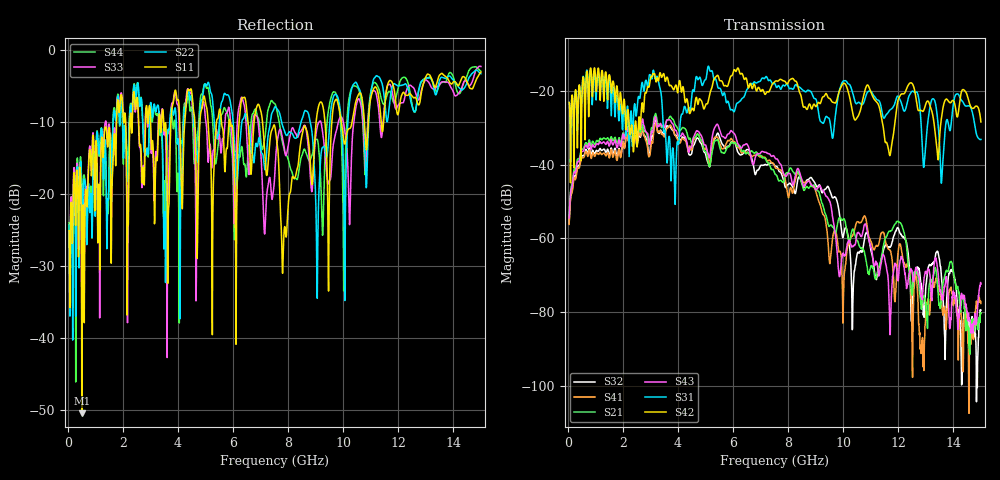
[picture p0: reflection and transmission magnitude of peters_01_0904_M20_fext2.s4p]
# MHZ S RI R 50.00
! FREQ  S11  S12  S13  S14
!  S21  S22  S23  S24
!  S31  S32  S33  S34
!  S41  S42  S43  S44
!  REAL  IMAG  REAL  IMAG  REAL  IMAG  REAL  IMAG
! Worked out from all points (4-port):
!   1496 points, 50 MHz to 15 GHz, reference 50 ohm
!   strongest paths, dB at 50 MHz, 3.79 GHz, 7.53 GHz, 11.27 GHz, 15 GHz:
!     S42: -23.1, -19.0, -17.4, -23.6, -28.4
!     S31: -23.1, -36.8, -18.2, -22.5, -33.2
!     S43: -54.4, -28.8, -38.2, -69.1, -72.4
!     S21: -53.7, -27.5, -42.6, -68.4, -80.2
!     S41: -56.2, -30.1, -40.8, -61.9, -77.7
!     S32: -55.9, -30.6, -40.4, -68.5, -79.5
!   lowest |S11| = -50.5 dB at 510 MHz (marker M1), VSWR 1.01, Z = 50.3 + j0.141 ohm
!   |S11| at or under -10 dB: start of sweep to 1.771 GHz; 7.073 GHz to 9.016 GHz (1.943 GHz wide, 24.2 % of centre); 9.935 GHz to 10.32 GHz (386.3 MHz wide, 3.81 % of centre)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
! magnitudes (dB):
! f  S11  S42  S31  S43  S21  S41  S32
! 50 MHz  -25.1  -23.1  -23.1  -54.4  -53.7  -56.2  -55.9
! 510 MHz  -50.5  -23.7  -21.9  -36.5  -35.8  -38.2  -37.8
! 3.16 GHz  -23.5  -15.5  -16.4  -27.5  -26.8  -29.6  -28.8
! 3.88 GHz  -5.9  -19.1  -46.2  -30.4  -28.9  -31.7  -31.9
! 5.46 GHz  -9.4  -15.9  -19.2  -29.3  -33.5  -32.8  -31.5
! 7.84 GHz  -26.3  -17.3  -18.5  -42.5  -44.7  -42.8  -44.3
! 15 GHz  -3.0  -28.4  -33.2  -72.4  -80.2  -77.7  -79.5
